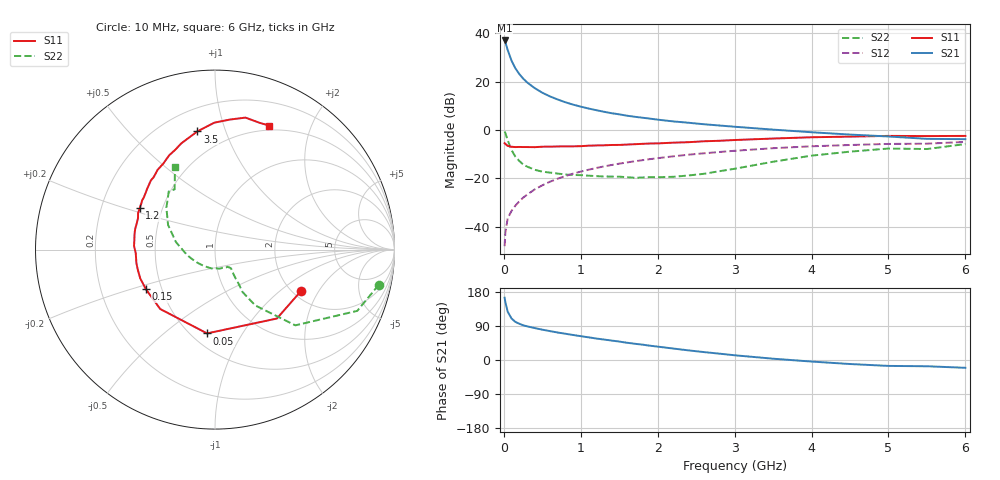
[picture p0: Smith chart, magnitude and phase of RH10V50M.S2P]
! SIEMENS Small Signal Semiconductors
! BFR106
! Si NPN RF Bipolar Junction Transistor in SOT23
! VCE = 10 V  IC = 50 mA
! Common Emitter S-Parameters:  August  1996
# GHz  S  MA  R  50
!  f  S11  S21  S12  S22
! GHz  MAG  ANG  MAG  ANG  MAG  ANG  MAG  ANG
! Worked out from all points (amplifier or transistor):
!   36 points, 10 MHz to 6 GHz, reference 50 ohm
!   highest |S21| = 36.9 dB at 10 MHz (marker M1)
!   |S21| within 3 dB of that: start of sweep to 41.2 MHz
!   unconditionally stable (mu >= 1): 267.9 MHz to 2.286 GHz
!   at 250 MHz: K = 0.99, MSG = 24.6 dB, |S12| = -28.0 dB
!   at 1.4 GHz: K = 1.06, MAG = 9.1 dB, |S12| = -14.5 dB
!   at 6 GHz: K = 0.98, MSG = 0.6 dB, |S12| = -4.9 dB
!   S11 on the Smith chart (normalised r, x): 10 MHz: 2.23, -1.42; 50 MHz: 0.60, -0.71; 150 MHz: 0.41, -0.23; 1.2 GHz: 0.37, +0.22; 3.5 GHz: 0.34, +0.80; 6 GHz: 0.45, +1.43
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0.01  0.5326 -25.4  70.38 164.4  0.004 82.4  0.9335 -12.1
0.02  0.516 -48.1  64.65 152.3  0.0077 74.2  0.8631 -23.3
0.05  0.469 -95.4  44.72 127.4  0.015 60.8  0.6153 -43.3
0.1  0.4503 -132.7  26.92 109.5  0.0214 59.8  0.3839 -54.2
0.15  0.4438 -150.1  18.7 100.6  0.0275 62.0  0.2816 -57.0
0.2  0.4463 -158.9  14.34 95.7  0.0335 65.2  0.2304 -55.3
0.25  0.4446 -165.6  11.53 91.7  0.04 67.0  0.1946 -54.3
0.3  0.4443 -170.3  9.666 89.0  0.0459 69.0  0.1764 -53.4
0.4  0.4419 -177.4  7.33 84.3  0.0593 70.3  0.1511 -51.0
0.5  0.4516 177.4  5.874 80.1  0.0721 71.1  0.1379 -49.6
0.6  0.453 172.4  4.928 76.2  0.0856 70.8  0.1321 -50.2
0.7  0.4568 168.9  4.257 72.5  0.0988 70.3  0.1261 -51.8
0.9  0.4595 162.0  3.336 66.0  0.1256 68.4  0.1177 -54.2
1.1  0.4742 154.7  2.775 59.8  0.1511 66.4  0.1142 -61.6
1.2  0.4792 151.1  2.564 56.8  0.1641 65.3  0.1114 -64.8
1.6  0.5002 140.4  1.971 45.6  0.2137 60.0  0.1062 -82.9
2.2  0.5472 125.8  1.504 30.3  0.2858 52.0  0.108 -118.5
2.8  0.5987 111.7  1.238 16.8  0.3511 43.4  0.1407 -159.3
3.5  0.6659 98.5  1.017 3.4  0.4206 33.5  0.2212 169.2
4.5  0.7298 83.3  0.804 -10.6  0.4898 18.8  0.3572 139.3
5.5  0.7488 70.4  0.656 -16.5  0.5215 8.5  0.4043 123.8
6  0.7542 66.4  0.646 -20.6  0.5668 1.5  0.5122 115.8
